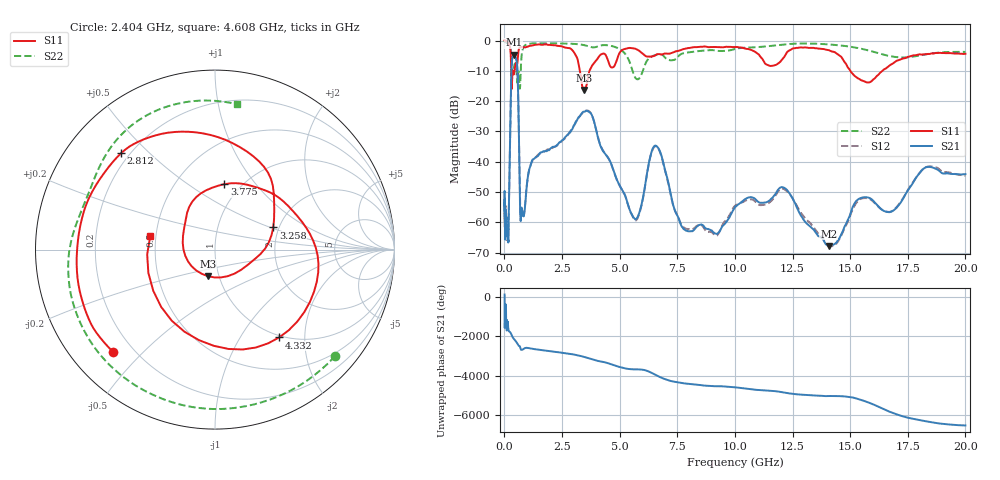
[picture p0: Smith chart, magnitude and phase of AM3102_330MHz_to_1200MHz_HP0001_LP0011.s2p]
! Date/Time: Tue, Sep 11, 2018 5:09 PM
! Network Analyzer: Agilent Technologies E8362B Rev: A.07.50.63
! Sweep from 0.010 to 20.000 GHz, 1601 Points, Sweep Type: LOG
! Power Supply: 4.950 V, 0.001 A
# Hz S DB R 50
!freq MagS11 AngS11 MagS21 AngS21 MagS12 AngS12 MagS22 AngS22
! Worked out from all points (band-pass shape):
!   1601 points, 10 MHz to 20 GHz, reference 50 ohm
!   highest |S21| = -4.70 dB at 406.7 MHz (marker M1); lowest = -67.8 dB at 14.07 GHz (marker M2)
!   |S21| within 3 dB of the highest: 318.8 MHz to 547.8 MHz (229 MHz wide, 52.9 % of centre)
!   lowest |S11| = -16.3 dB at 3.449 GHz (marker M3), VSWR 1.36, Z = 44.3 - j13.4 ohm
!   |S11| at or under -10 dB: 295.6 MHz to 362.6 MHz (67.03 MHz wide, 20.4 % of centre); 3.28 GHz to 3.694 GHz (414.8 MHz wide, 11.9 % of centre); 15.01 GHz to 16.4 GHz (1.393 GHz wide, 8.87 % of centre)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
!   |S22| runs from -15.9 to -0.2 dB; largest |S21 - S12| = 0.0092
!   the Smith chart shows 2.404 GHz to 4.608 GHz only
!   S11 on the Smith chart (normalised r, x): 2.404 GHz: 0.13, -0.41; 2.812 GHz: 0.17, +0.41; 3.258 GHz: 1.86, +0.52; 3.775 GHz: 0.84, +0.71; 4.332 GHz: 0.97, -1.50; 4.608 GHz: 0.47, +0.08
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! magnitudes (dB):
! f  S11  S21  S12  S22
! 10 MHz  0.0  -50.0  -50.2  -0.2
! 35.55 MHz  0.0  -64.6  -59.6  -0.4
! 126.4 MHz  -0.4  -62.6  -63.0  -0.9
! 172.1 MHz  -0.8  -66.0  -62.8  -1.1
! 406.7 MHz  -11.2  -4.7  -4.8  -9.1
! 447.2 MHz  -9.3  -5.0  -5.1  -7.7
! 572.5 MHz  -6.8  -11.0  -11.1  -13.4
! 702.3 MHz  -2.2  -59.3  -59.1  -11.7
! 1.59 GHz  -1.4  -36.9  -37.0  -0.9
! 2.404 GHz  -1.9  -33.5  -33.8  -1.0
! 2.812 GHz  -2.5  -30.5  -30.5  -1.0
! 3.258 GHz  -9.2  -25.1  -25.1  -1.3
! 3.449 GHz  -16.3  -23.5  -23.5  -1.5
! 3.775 GHz  -8.7  -24.3  -24.3  -2.2
! 4.332 GHz  -4.3  -36.9  -36.9  -1.5
! 4.608 GHz  -8.7  -40.2  -40.3  -1.7
! 5.652 GHz  -2.7  -58.8  -59.2  -11.9
! 6.58 GHz  -4.7  -34.7  -34.9  -4.8
! 7.882 GHz  -2.6  -62.8  -62.1  -4.0
! 12.03 GHz  -6.4  -48.4  -48.9  -1.4
! 14.07 GHz  -3.2  -67.8  -67.7  -1.3
! 20 GHz  -4.4  -44.1  -44.6  -3.7
